ORGANIZATION_BLOCK "RACK_FLT"
TITLE = "Loss Of Rack Fault"
VERSION : 0.1


VAR_TEMP
  OB86_EV_CLASS : BYTE ;	//16#38/39 Event class 3
  OB86_FLT_ID : BYTE ;	//16#C1/C4/C5, Fault identifcation code
  OB86_PRIORITY : BYTE ;	//Priority of OB Execution
  OB86_OB_NUMBR : BYTE ;	//86 (Organization block 86, OB86)
  OB86_RESERVED_1 : BYTE ;	//Reserved for system
  OB86_RESERVED_2 : BYTE ;	//Reserved for system
  OB86_MDL_ADDR : WORD ;	//Base address of IM module in rack with fault
  OB86_RACKS_FLTD : ARRAY  [0 .. 31 ] OF BOOL ;	//Racks in fault
  OB86_DATE_TIME : DATE_AND_TIME ;	//Date and time OB86 started
END_VAR
BEGIN
END_ORGANIZATION_BLOCK

